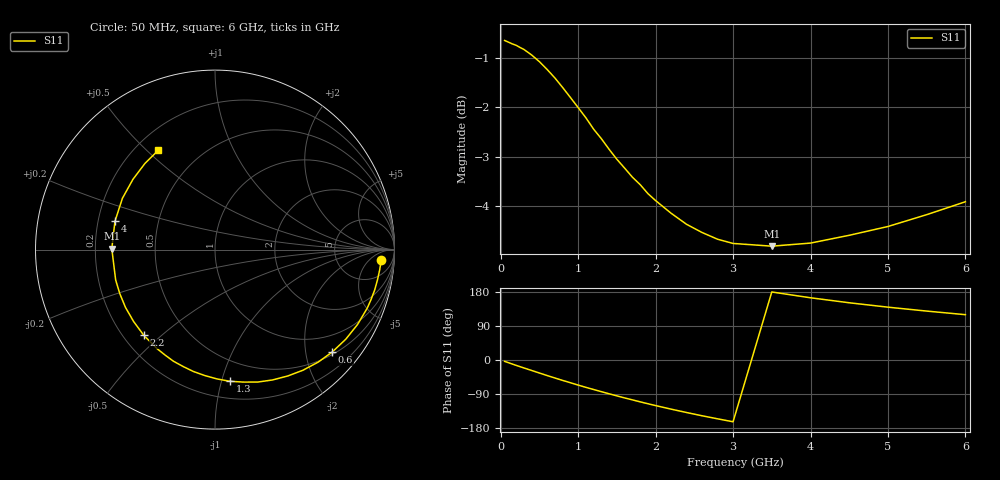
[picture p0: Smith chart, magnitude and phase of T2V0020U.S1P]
! SIEMENS Discrete & RF Semiconductors
! BAS70-04W
! Si Schottky Diode in SOT323
! IF = 0.02 mA
! S-Parameters:  November  1997
# GHz  S  MA  R  50
!  f  S11
! GHz  MAG  ANG
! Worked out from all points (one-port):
!   34 points, 50 MHz to 6 GHz, reference 50 ohm
!   lowest |S11| = -4.8 dB at 3.5 GHz (marker M1), VSWR 3.71, Z = 13.5 + j0.202 ohm
!   |S11| at or under -10 dB: nowhere
!   S11 on the Smith chart (normalised r, x): 50 MHz: 16, -13; 600 MHz: 0.56, -2.56; 1.3 GHz: 0.33, -1.06; 2.2 GHz: 0.28, -0.44; 4 GHz: 0.27, +0.13; 6 GHz: 0.29, +0.54
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0.05  0.9281 -3.6
0.2  0.9176 -14.2
0.3  0.9088 -21.0
0.4  0.8972 -27.7
0.5  0.8833 -34.4
0.6  0.8674 -41.1
0.7  0.8505 -47.5
0.8  0.8318 -53.9
0.9  0.8127 -60.0
1  0.7938 -66.2
1.1  0.7752 -72.2
1.3  0.7383 -83.6
1.4  0.7203 -89.2
1.6  0.6895 -100.1
1.8  0.6636 -110.4
1.9  0.6499 -115.4
2  0.6394 -120.3
2.2  0.6208 -129.7
2.4  0.605 -138.6
2.6  0.5936 -147.2
2.8  0.5844 -155.2
3  0.5787 -163.0
3.5  0.575 179.5
4  0.5792 164.2
4.5  0.5898 151.0
5  0.602 139.4
5.5  0.6188 129.1
6  0.6377 119.6
